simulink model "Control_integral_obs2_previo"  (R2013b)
settings: Solver=ode45  StartTime=0.0  StopTime=0.025  MaxStep=1e-4  RelTol=1e-3
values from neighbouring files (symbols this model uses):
  Am = [-R1/L1 R1/L1; R1/L2 -(R1+R2)/L2]    [Clase_25_11_2021.m]
  Bm = [-1/L1;0]    [Clase_25_11_2021.m]
  Lo1 = L(1)    [Clase_25_11_2021.m]
  Lo2 = L(2)    [Clase_25_11_2021.m]
  R2 = 5    [Clase_25_11_2021.m]

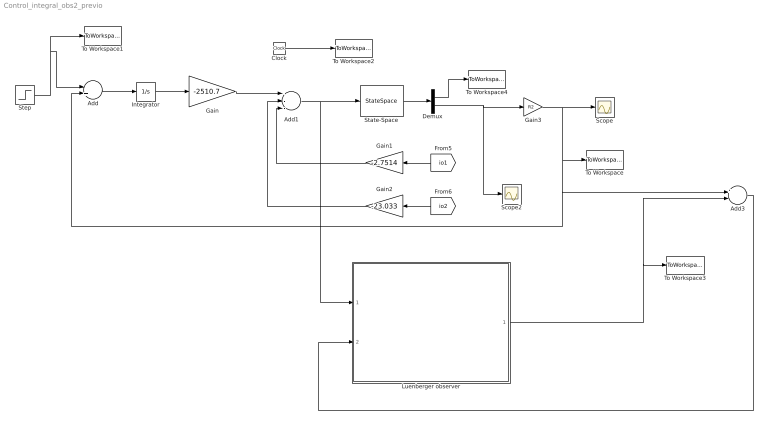
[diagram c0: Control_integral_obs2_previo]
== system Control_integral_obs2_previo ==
  Add : Sum  Inputs=-+
  Add1 : Sum  Inputs=---
  Add3 : Sum  Inputs=+-
  Clock : Clock
  Demux : Demux  Outputs=2
  Gain : Gain  Gain=-2510.7
  Gain1 : Gain  Gain=-2.7514
  Gain2 : Gain  Gain=-23.033
  Gain3 : Gain  Gain=R2
  Integrator : Integrator
  Luenberger observer : Subsystem
  Scope : Scope
  Scope2 : Scope
  State-Space : StateSpace  A=Am  B=Bm  C=[1 0;0 1]  D=[0;0]  X0=0
  Step : Step  Time=0.01  After=50  SampleTime=0
  To Workspace : ToWorkspace  VariableName=E  SampleTime=-1
  To Workspace1 : ToWorkspace  VariableName=in  SampleTime=-1
  To Workspace2 : ToWorkspace  VariableName=time  SampleTime=-1
  To Workspace3 : ToWorkspace  VariableName=Eo  SampleTime=-1
  To Workspace4 : ToWorkspace  VariableName=i1  SampleTime=-1
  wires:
  Step/1 -> To Workspace1/1, Add/1
  Add/1 -> Integrator/1
  Integrator/1 -> Gain/1
  Gain/1 -> Add1/1
  Add1/1 -> Luenberger observer/1(Excitacion U), State-Space/1
  State-Space/1 -> Demux/1
  Demux/2 -> Gain3/1, Scope2/1
  Gain1/1 -> Add1/3
  Gain2/1 -> Add1/2
  Gain3/1 -> Add/2, Add3/1, To Workspace/1, Scope/1
  Clock/1 -> To Workspace2/1
  Add3/1 -> Luenberger observer/2((Y-Yo))
  Luenberger observer/1(Eo) -> To Workspace3/1, Add3/2
  Demux/1 -> To Workspace4/1
  [io1] -> Gain1/1
  [io2] -> Gain2/1

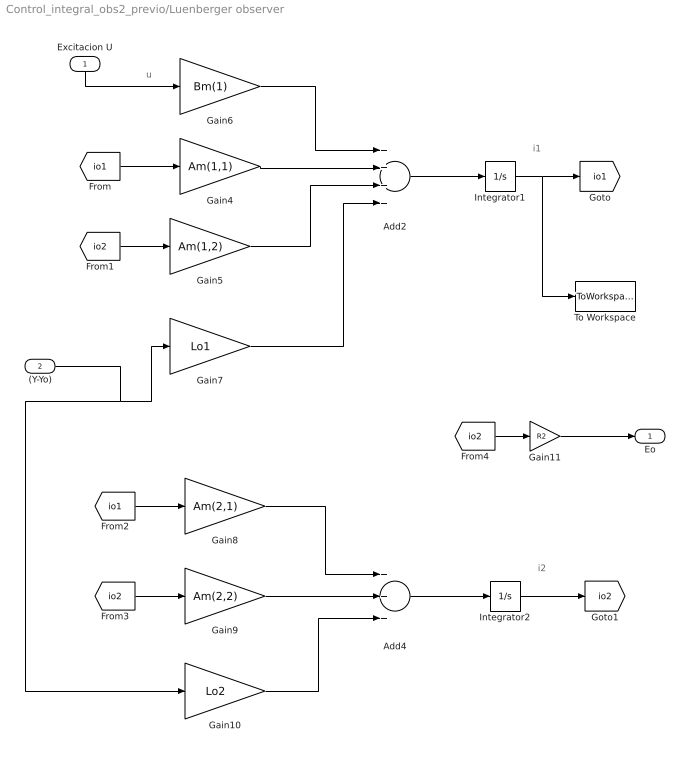
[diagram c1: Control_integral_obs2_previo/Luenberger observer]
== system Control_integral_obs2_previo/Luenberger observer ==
  note: u
  note: i1
  note: i2
  Excitacion U : Inport
  (Y-Yo) : Inport  Port=2
  Add2 : Sum  Inputs=++++
  Add4 : Sum  Inputs=+++
  Gain10 : Gain  Gain=Lo2
  Gain11 : Gain  Gain=R2
  Gain4 : Gain  Gain=Am(1,1)
  Gain5 : Gain  Gain=Am(1,2)
  Gain6 : Gain  Gain=Bm(1)
  Gain7 : Gain  Gain=Lo1
  Gain8 : Gain  Gain=Am(2,1)
  Gain9 : Gain  Gain=Am(2,2)
  Integrator1 : Integrator
  Integrator2 : Integrator
  To Workspace : ToWorkspace  VariableName=io1  SampleTime=-1
  Eo : Outport
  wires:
  Gain6/1 -> Add2/1
  Gain7/1 -> Add2/4
  Add2/1 -> Integrator1/1
  Gain8/1 -> Add4/1
  Integrator2/1 -> [io2]
  (Y-Yo)/1 -> Gain10/1, Gain7/1
  Gain11/1 -> Eo/1
  [io2] -> Gain11/1
  Gain10/1 -> Add4/3
  Add4/1 -> Integrator2/1
  [io1] -> Gain8/1
  [io2] -> Gain9/1
  [io2] -> Gain5/1
  Integrator1/1 -> To Workspace/1, [io1]
  Gain9/1 -> Add4/2
  [io1] -> Gain4/1
  Excitacion U/1 -> Gain6/1
  Gain5/1 -> Add2/3
  Gain4/1 -> Add2/2
